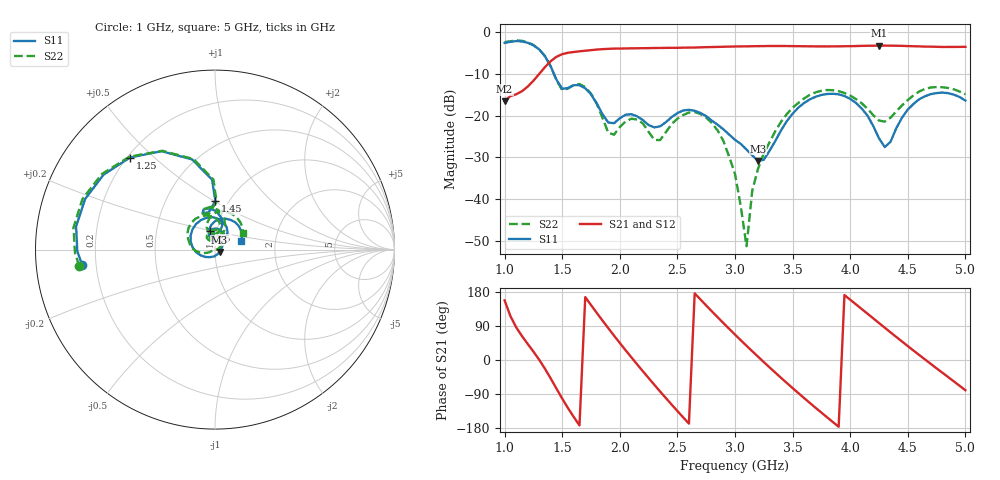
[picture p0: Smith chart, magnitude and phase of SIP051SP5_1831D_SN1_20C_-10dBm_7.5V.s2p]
# GHz  S  dB  R  50
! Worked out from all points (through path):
!   81 points, 1 GHz to 5 GHz, reference 50 ohm
!   highest |S21| = -3.18 dB at 4.25 GHz (marker M1); lowest = -16.5 dB at 1 GHz (marker M2)
!   lowest |S11| = -30.8 dB at 3.2 GHz (marker M3), VSWR 1.06, Z = 52.6 - j1.41 ohm
!   |S11| at or under -10 dB: 1.429 GHz to end of sweep
!   |S22| runs from -51.2 to -2.0 dB; largest |S21 - S12| = 0.0024
!   S11 on the Smith chart (normalised r, x): 1 GHz: 0.15, -0.05; 1.25 GHz: 0.21, +0.42; 1.45 GHz: 0.87, +0.51; 2.5 GHz: 0.93, +0.20; 5 GHz: 1.33, +0.12
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1  -2.55 -173.6  -16.52 157.3  -16.51 157.1  -2.36 -173.0
1.25  -3.12 132.7  -11.62 22.2  -11.60 22.2  -3.06 132.6
1.45  -11.34 89.5  -5.87 -75.4  -5.87 -75.3  -11.48 88.2
1.55  -13.35 108.7  -4.91 -126.9  -4.91 -126.7  -13.48 108.9
1.7  -13.41 87.9  -4.42 166.0  -4.43 165.9  -13.12 85.2
1.9  -21.62 86.5  -3.97 84.0  -3.96 84.0  -24.07 76.3
2.1  -19.62 99.4  -3.85 7.2  -3.84 7.1  -20.71 100.4
2.35  -22.53 107.7  -3.76 -83.1  -3.76 -83.2  -25.82 114.4
2.5  -19.38 104.4  -3.73 -134.6  -3.71 -134.6  -20.70 118.4
2.7  -19.33 69.6  -3.61 159.8  -3.61 159.8  -19.57 77.1
2.85  -22.17 48.4  -3.51 112.7  -3.51 112.6  -23.55 45.9
3  -25.77 33.6  -3.41 67.0  -3.40 67.1  -33.93 17.6
3.1  -28.09 14.8  -3.37 37.6  -3.37 37.5  -51.24 -121.8
3.15  -29.50 -1.5  -3.35 23.0  -3.34 23.1  -37.89 -157.4
3.2  -30.82 -27.8  -3.33 8.8  -3.33 8.7  -32.69 -157.0
3.45  -21.28 -158.1  -3.30 -60.7  -3.30 -60.7  -19.60 -175.0
3.7  -15.45 137.8  -3.38 -126.2  -3.39 -126.2  -14.39 140.6
3.95  -15.27 82.9  -3.35 171.4  -3.35 171.4  -14.54 96.9
4.25  -25.40 53.0  -3.18 97.5  -3.20 97.7  -21.15 85.5
4.35  -26.25 102.2  -3.22 73.0  -3.21 73.0  -20.48 106.6
4.65  -15.34 81.3  -3.44 1.3  -3.43 1.2  -13.55 87.2
5  -16.36 17.4  -3.49 -79.7  -3.50 -79.7  -14.87 30.4
